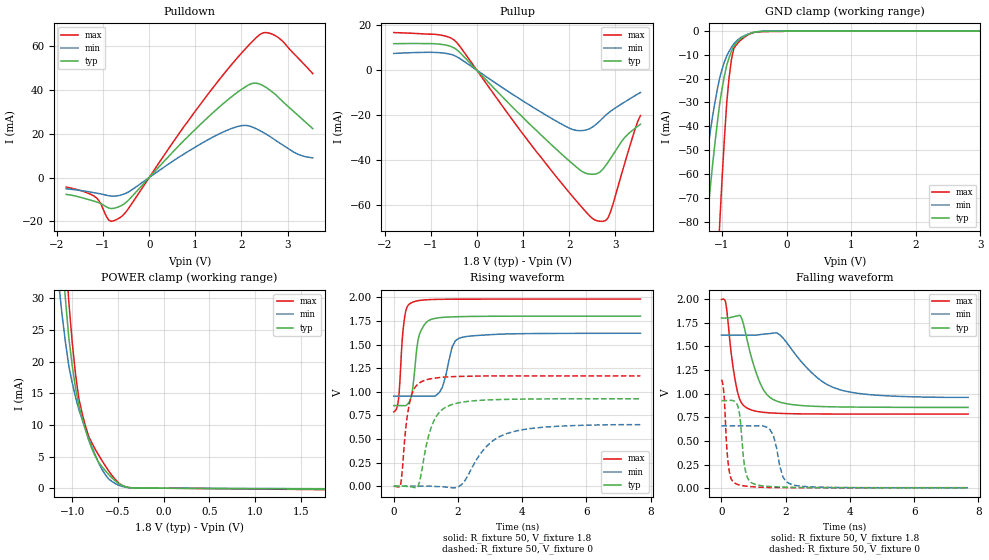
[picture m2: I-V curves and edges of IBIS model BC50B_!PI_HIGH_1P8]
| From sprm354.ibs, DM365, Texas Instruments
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|   Model Cell BC50B_!PI_HIGH_1P8
|BC1833DV50BTHYPBFZP_!PI_HIGH_1P8
[Model]   BC50B_!PI_HIGH_1P8
Model_type   I/O
Polarity   Non-Inverting
Enable   Active-Low
Vinl =  0.63V
Vinh =  1.17V
Cref =  15pF
Rref =  100.00M
Vref =  0V
Vmeas =  0.9
C_comp   1.889253p   1.773057p   1.933707p
[Model Spec]
Vinl   0.63V   0.567V   0.693V
Vinh   1.17V   1.053V   1.287V
[Temperature Range]   25   125   -40
[Voltage Range]   1.8   1.62   1.98
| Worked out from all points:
|   slope of the pulldown table from 0 to 0.27 V, typ, clamps not added: 43.6 ohm
|   slope of the pullup table from 0 to 0.27 V, typ, clamps not added: 46.6 ohm
|   GND clamp passes 1 mA (typ) near -0.55 V on its own axis
|   POWER clamp passes 1 mA (typ) near -0.52 V on its own axis
|   rising waveform, R_fixture 50, V_fixture 1.8: 20-80 % time 210ps typ, 289ps min, 146ps max; typ from 0.854 V to 1.8 V
|   rising waveform, R_fixture 50, V_fixture 0: 20-80 % time 445ps typ, 939ps min, 248ps max; typ from 0.003 V to 0.926 V
|   falling waveform, R_fixture 50, V_fixture 1.8: 20-80 % time 532ps typ, 1.17ns min, 289ps max; typ from 1.8 V to 0.854 V
|   falling waveform, R_fixture 50, V_fixture 0: 20-80 % time 167ps typ, 260ps min, 127ps max; typ from 0.926 V to 0.003 V
[POWER_clamp]
|   voltage   I(typ)   I(min)   I(max)
-1.8V     212.5mA    175.3mA    247.1mA
-1.145V   43.74mA    32.23mA    55.31mA
-1.109V   36.46mA    27.32mA    46.17mA
-1.073V   29.8mA     23.02mA    37.55mA
-1.036V   23.79mA    19.34mA    29.46mA
-963.6mV  15.92mA    14.44mA    18.12mA
-927.3mV  13.11mA    12.48mA    14.23mA
-854.5mV  9.226mA    9.295mA    9.82mA
-672.7mV  3.38mA     2.951mA    4.34mA
-527.3mV  1.139mA    717.2uA    1.363mA
-345.5mV  64.92uA    52.08uA    68.3uA
1.764V    -147uA     -80.5uA    -230.4uA
[Pulldown]
|   voltage   I(typ)   I(min)   I(max)
-1.8V     -7.67mA    -5.126mA   -4.339mA
-1.145V   -11.1mA    -7.106mA   -9.219mA
-872.7mV  -13.94mA   -8.311mA   -19.49mA
-600mV    -12.75mA   -7.913mA   -17.78mA
763.6mV   17.11mA    10.84mA    23.53mA
1.636V    34.26mA    21.05mA    47.69mA
2.182V    42.48mA    23.41mA    60.84mA
2.455V    42.04mA    20.75mA    65.84mA
2.618V    39.8mA     18.68mA    65.73mA
2.836V    35.82mA    15.63mA    63.15mA
3.218V    28.47mA    10.66mA    54.66mA
3.545V    22.28mA    8.953mA    47.39mA
[Pullup]
|   voltage   I(typ)   I(min)   I(max)
-1.8V     11.79mA    7.463mA    16.74mA
-872.7mV  11.71mA    7.882mA    15.87mA
-490.9mV  9.875mA    6.533mA    13.41mA
981.8mV   -20.64mA   -13.44mA   -27.9mA
1.964V    -39.57mA   -25.31mA   -53.36mA
2.291V    -45.08mA   -26.79mA   -61.23mA
2.564V    -46.14mA   -24.37mA   -66.57mA
2.782V    -42.64mA   -20.2mA    -66.89mA
2.891V    -39.37mA   -18.32mA   -63.27mA
3.218V    -29.56mA   -13.93mA   -40.37mA
3.436V    -25.67mA   -11.18mA   -25.75mA
3.545V    -23.99mA   -9.92mA    -20.12mA
[GND_clamp]
|   voltage   I(typ)   I(min)   I(max)
-1.8V     -250.5mA   -178.5mA   -583.5mA
-1.4V     -128mA     -86.67mA   -313.9mA
-1.364V   -117.2mA   -78.73mA   -289.5mA
-1.255V   -85.5mA    -55.96mA   -216.9mA
-1.218V   -75.35mA   -48.88mA   -193mA
-1.036V   -30.44mA   -19.69mA   -80.61mA
-963.6mV  -18.83mA   -13.02mA   -45.03mA
-890.9mV  -11.2mA    -8.571mA   -19.45mA
-818.2mV  -6.355mA   -5.478mA   -7.373mA
-709.1mV  -3.264mA   -2.787mA   -3.874mA
-18.18mV  0A         0A         0A
3.6V      0A         0A         0A
[Ramp]
| variable   typ   min   max
dV/dt_f  0.5852885/0.5373076n  0.4137874/1.206677n   0.7298059/0.2885627n
dV/dt_r  0.5660011/0.4440676n  0.4050825/0.966649n   0.7053755/0.247472n
R_load = 50
[Rising Waveform]
R_fixture = 50
V_fixture = 1.8
V_fixture_min = 1.62
V_fixture_max = 1.98
|   time   V(typ)   V(min)   V(max)
0s        854.3mV    955mV      787.2mV
150ps     854.3mV    955mV      932.4mV
342ps     852.5mV    955mV      1.8V
558ps     971.6mV    955mV      1.943V
756ps     1.552V     955mV      1.964V
1.152ns   1.764V     954.7mV    1.975V
1.512ns   1.787V     1.048V     1.978V
1.812ns   1.792V     1.47V      1.979V
2.112ns   1.795V     1.575V     1.98V
7.68ns    1.8V       1.619V     1.98V
[Rising Waveform]
R_fixture = 50
V_fixture = 0
V_fixture_min = 0
V_fixture_max = 0
|   time   V(typ)   V(min)   V(max)
0s        3.475mV    2.101mV    711.1uV
216ps     3.525mV    2.104mV    25.74mV
384ps     -592.8uV   2.101mV    651.6mV
516ps     -4.301mV   2.096mV    921.7mV
756ps     1.933mV    2.089mV    1.082V
912ps     248.6mV    2.098mV    1.115V
1.272ns   709.6mV    -969.4uV   1.144V
1.812ns   864.9mV    -15.28mV   1.16V
3.492ns   919.6mV    555.2mV    1.168V
7.68ns    926.3mV    652.3mV    1.168V
[Falling Waveform]
R_fixture = 50
V_fixture = 1.8
V_fixture_min = 1.62
V_fixture_max = 1.98
|   time   V(typ)   V(min)   V(max)
0s        1.8V       1.62V      1.997V
126ps     1.8V       1.62V      1.971V
492ps     1.823V     1.62V      1.029V
636ps     1.791V     1.62V      896.2mV
834ps     1.516V     1.62V      841.2mV
1.272ns   1.063V     1.629V     804.1mV
1.812ns   910.8mV    1.625V     791.6mV
2.91ns    866.1mV    1.19V      785.2mV
3.678ns   859.6mV    1.043V     784.6mV
7.68ns    854.5mV    960.9mV    784.5mV
[Falling Waveform]
R_fixture = 50
V_fixture = 0
V_fixture_min = 0
V_fixture_max = 0
|   time   V(typ)   V(min)   V(max)
0s        926.4mV    658.7mV    1.149V
84ps      926.3mV    658.7mV    966.4mV
234ps     926.9mV    658.7mV    196.9mV
474ps     894.1mV    658.8mV    43.23mV
756ps     167.4mV    658.8mV    21.16mV
1.032ns   41.94mV    659.2mV    13.42mV
1.512ns   17.43mV    618.5mV    7.247mV
1.914ns   11.22mV    116mV      5.726mV
2.214ns   8.419mV    35.88mV    5.318mV
7.68ns    3.491mV    3.045mV    5.001mV
